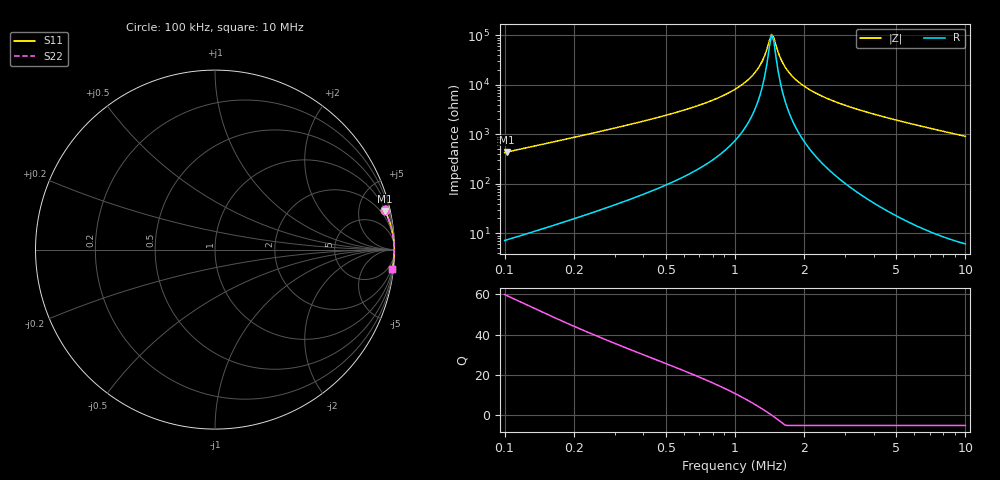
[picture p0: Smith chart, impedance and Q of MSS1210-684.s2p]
# MHz S MA R 50
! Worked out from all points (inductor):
!   203 points, 100 kHz to 10 MHz, reference 50 ohm
!   read as one part in series: L = 680 uH near 102.3 kHz
!   highest Q = 59.4 at 102.3 kHz (marker M1), where L = 683 uH
!   self-resonance near 1.44 MHz
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0.1  0.9703 13.1  0.226 -76.0  0.226 -76.0  0.9703 13.1
0.102306  0.9715 12.8  0.2212 -76.3  0.2212 -76.3  0.9715 12.8
0.1981663  0.9908 6.6  0.1149 -82.1  0.1149 -82.1  0.9908 6.6
0.3424944  0.996 3.7  0.0643 -84.6  0.0643 -84.6  0.996 3.7
0.97746  0.9988 0.7  0.01306 -84.2  0.01306 -84.2  0.9988 0.7
1.173024  0.9989 0.4  0.006917 -80.9  0.006917 -80.9  0.9989 0.4
1.256059  0.999 0.3  0.004702 -77.4  0.004702 -77.4  0.999 0.3
1.314655  0.999 0.2  0.00326 -72.2  0.00326 -72.2  0.999 0.2
1.375986  0.999 0.1  0.001893 -59.3  0.001893 -59.3  0.999 0.1
1.440177  0.9991 0.0  0.0009553 -9.3  0.0009553 -9.3  0.9991 0.0
1.473387  0.9991 -0.0  0.001099 32.0  0.001099 32.0  0.9991 -0.0
1.542122  0.9991 -0.1  0.002251 66.0  0.002251 66.0  0.9991 -0.1
1.614064  0.9991 -0.2  0.003649 75.6  0.003649 75.6  0.9991 -0.2
1.768173  0.9991 -0.4  0.00658 82.2  0.00658 82.2  0.9991 -0.4
1.981663  0.9991 -0.6  0.01037 84.9  0.01037 84.9  0.9991 -0.6
2.324538  0.9991 -0.9  0.01593 86.4  0.01593 86.4  0.9991 -0.9
2.789617  0.999 -1.3  0.02279 86.9  0.02279 86.9  0.999 -1.3
3.424944  0.9989 -1.8  0.03144 87.0  0.03144 87.0  0.9989 -1.8
5.162633  0.998 -3.0  0.0531 86.3  0.0531 86.3  0.998 -3.0
6.787083  0.9968 -4.1  0.07222 85.4  0.07222 85.4  0.9968 -4.1
8.524974  0.9951 -5.3  0.09214 84.3  0.09214 84.3  0.9951 -5.3
10  0.9933 -6.2  0.1088 83.4  0.1088 83.4  0.9933 -6.2
